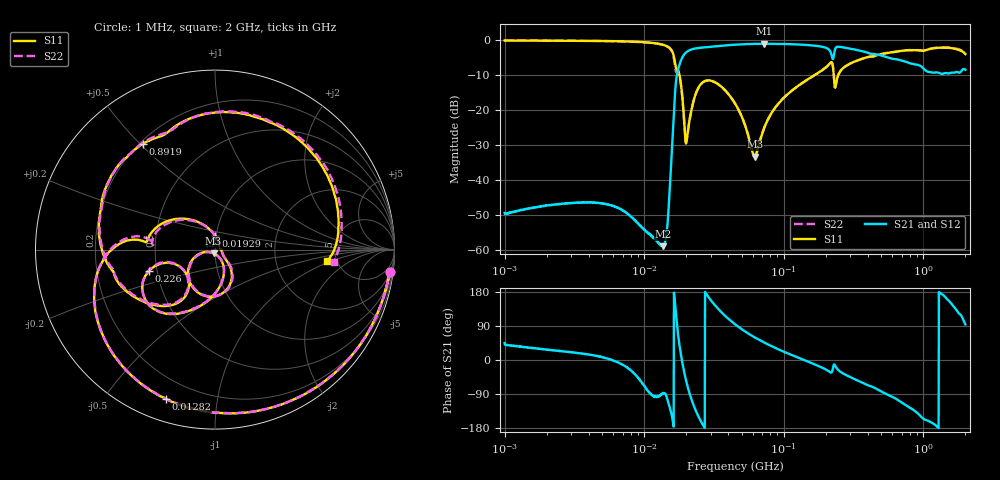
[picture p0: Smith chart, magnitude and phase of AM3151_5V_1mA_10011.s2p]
! Date/Time: Fri Jun 26 10:53:33 2020
! Network Analyzer:  Rev:
! Sweep from 1000000.0 to 2000000000.0, 1601 Points ! Power Supply: 0 V, 0 A
# HZ S DB R 50
!freq MagS11 AngS11 MagS21 AngS21 MagS12 AngS12 MagS22 AngS22
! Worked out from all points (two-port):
!   1601 points, 1 MHz to 2 GHz, reference 50 ohm
!   highest |S21| = -1.11 dB at 72.26 MHz (marker M1); lowest = -59.0 dB at 13.64 MHz (marker M2)
!   |S21| within 3 dB of the highest: 19.38 MHz to 219 MHz (199.6 MHz wide, 167 % of centre); 229.1 MHz to 459.3 MHz (230.2 MHz wide, 66.9 % of centre)
!   lowest |S11| = -33.4 dB at 62.07 MHz (marker M3), VSWR 1.04, Z = 49.2 - j1.97 ohm
!   |S11| at or under -10 dB: 17.89 MHz to 167.1 MHz (149.2 MHz wide, 161 % of centre); 228 MHz to 245.7 MHz (17.77 MHz wide, 7.5 % of centre)
!   |S22| runs from -33.1 to -0.2 dB; largest |S21 - S12| = 0.0082
!   S11 on the Smith chart (normalised r, x): 1 MHz: 2, -15; 12.82 MHz: 0.10, -0.72; 19.29 MHz: 0.99, +0.15; 226 MHz: 0.45, -0.12; 891.9 MHz: 0.21, +0.51; 2 GHz: 4.16, -0.89
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1000000  -0.17 -7.4  -49.47 44.7  -49.76 40.0  -0.17 -7.5
3555161  -0.26 -25.7  -46.46 17.2  -46.45 16.8  -0.26 -25.7
7566571  -0.45 -56.2  -49.61 -20.8  -49.63 -20.0  -0.45 -56.4
1.263916e7  -1.09 -105.7  -57.88 -95.4  -57.96 -95.6  -1.12 -106.4
1.282058e7  -1.15 -108.0  -58.25 -93.6  -58.46 -95.4  -1.17 -108.7
1.363731e7  -1.39 -119.3  -58.96 -87.4  -58.91 -87.6  -1.43 -120.3
1.471428e7  -1.91 -137.6  -52.31 -106.1  -52.17 -105.7  -1.97 -139.2
1.696809e7  -8.15 173.8  -11.27 113.0  -11.26 112.9  -9.22 174.9
1.929026e7  -22.61 88.2  -4.20 -29.9  -4.20 -29.9  -22.86 86.0
2.022878e7  -28.39 -13.4  -3.39 -63.0  -3.39 -63.1  -28.10 -13.7
2.172285e7  -20.30 -44.7  -2.75 -101.9  -2.75 -102.0  -20.44 -42.8
2.639402e7  -12.07 -82.0  -2.18 -171.8  -2.18 -171.7  -12.11 -80.0
3.411262e7  -12.74 -127.1  -1.76 133.7  -1.74 133.7  -12.77 -125.6
4.493426e7  -18.29 -159.6  -1.35 93.8  -1.36 93.7  -18.35 -158.0
6.206852e7  -33.38 -110.9  -1.14 59.4  -1.15 59.4  -32.99 -108.7
7.225896e7  -25.29 -60.2  -1.11 46.2  -1.11 46.2  -25.15 -60.4
1.589914e8  -10.54 -99.8  -1.58 -8.5  -1.56 -8.6  -10.57 -100.1
2.259679e8  -8.30 -162.3  -5.33 -18.5  -5.34 -18.4  -8.20 -162.5
5.652395e8  -3.66 170.3  -5.11 -93.0  -5.08 -93.0  -3.65 168.2
8.918562e8  -2.94 124.3  -7.07 -137.7  -7.06 -137.8  -2.90 121.9
1.374171e9  -2.23 69.5  -9.70 172.5  -9.68 172.1  -2.17 67.1
2e9  -4.06 -5.9  -8.52 93.8  -8.69 93.5  -3.54 -5.9
